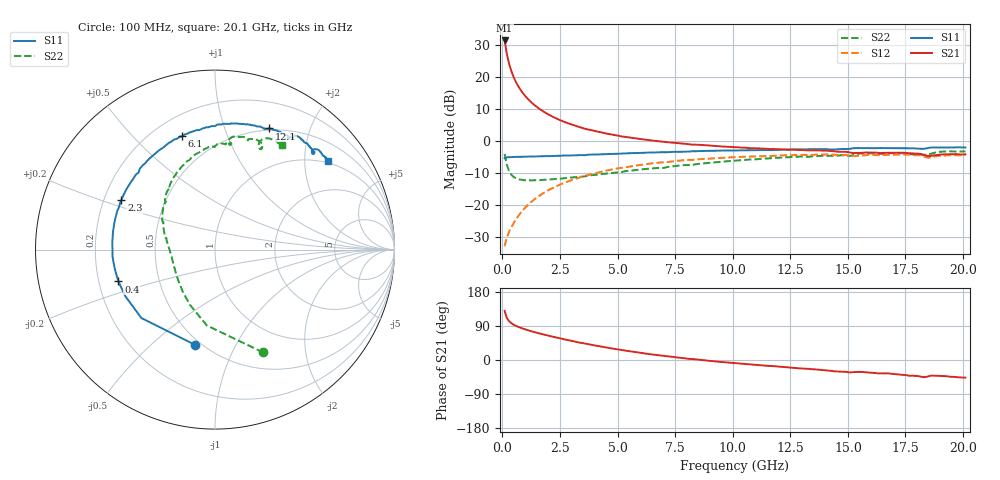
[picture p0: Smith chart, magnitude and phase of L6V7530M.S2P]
!  Infineon Technologies AG
! BFR380L3 , PF131585-7, No.6, Th 09.10.01, soldered on pcb-board, measured with PP GSG850
!  Vce=0.75 V,  Ic=30.0 mA
! Common Emitter S-Parameters:  15. November 2001
#  GHz  S  MA  R  50
! f  S11  S21  S12  S22
! GHz  Mag  Ang  Mag  Ang  Mag  Ang  Mag  Ang
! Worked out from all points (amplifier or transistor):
!   201 points, 100 MHz to 20.1 GHz, reference 50 ohm
!   highest |S21| = 31.6 dB at 100 MHz (marker M1)
!   |S21| within 3 dB of that: start of sweep to 169.4 MHz
!   unconditionally stable (mu >= 1): 1.011 GHz to 4.988 GHz; 5.179 GHz to 5.219 GHz; 18.31 GHz to 18.54 GHz
!   at 3.4 GHz: K = 1.02, MAG = 6.9 dB, |S12| = -11.2 dB
!   at 10.1 GHz: K = 0.98, MSG = 1.6 dB, |S12| = -5.0 dB
!   at 20.1 GHz: K = 0.99, MSG = 0.1 dB, |S12| = -4.3 dB
!   S11 on the Smith chart (normalised r, x): 100 MHz: 0.47, -0.70; 400 MHz: 0.28, -0.15; 2.3 GHz: 0.27, +0.23; 6.1 GHz: 0.31, +0.70; 12.1 GHz: 0.48, +1.43; 20.1 GHz: 0.94, +2.58
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0.1  0.5427 -101.6  37.88 129.7  0.02276 55.5  0.6329 -64.9
0.2  0.5602 -137.1  23.03 110.6  0.03143 52.3  0.425 -96.2
0.3  0.5631 -152.7  16.13 102.1  0.03843 54.9  0.3378 -114.4
0.4  0.5667 -161.8  12.33 96.7  0.04546 57.9  0.2965 -127.0
0.5  0.568 -168.0  9.955 92.8  0.05268 60.6  0.2749 -136.1
0.6  0.5697 -172.4  8.342 89.8  0.06035 62.3  0.2624 -143.0
0.7  0.5719 -176.2  7.191 87.1  0.06809 63.7  0.2551 -148.4
0.8  0.5715 -179.2  6.312 84.8  0.07591 64.7  0.2502 -152.9
1  0.5741 175.5  5.087 80.7  0.09186 65.5  0.2453 -159.6
1.2  0.5762 171.0  4.265 77.0  0.1078 65.7  0.2442 -164.6
1.5  0.5801 165.2  3.446 71.9  0.1317 65.1  0.2448 -170.6
1.9  0.5857 158.4  2.757 65.7  0.1634 63.2  0.2493 -176.5
2.3  0.5898 152.0  2.314 59.9  0.194 61.0  0.2564 178.4
3.5  0.6056 135.2  1.606 44.3  0.2818 52.4  0.2785 166.6
4.9  0.6354 118.6  1.244 28.9  0.3694 41.9  0.322 153.4
6.1  0.658 106.3  1.072 18.1  0.4315 33.1  0.3643 143.0
6.8  0.6711 99.8  0.9965 12.3  0.4631 27.8  0.3824 136.4
10.1  0.7186 75.9  0.8053 -8.4  0.5629 6.5  0.4972 112.1
12.1  0.7387 66.0  0.7475 -17.9  0.5988 -5.0  0.554 98.2
13.5  0.7478 59.4  0.7213 -24.4  0.6127 -12.9  0.581 89.5
16.8  0.7803 47.6  0.6599 -35.5  0.6136 -27.6  0.6495 71.6
20.1  0.7999 38.3  0.6263 -46.5  0.6063 -40.4  0.6952 57.3
